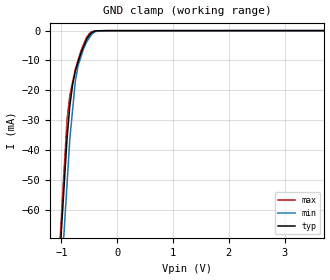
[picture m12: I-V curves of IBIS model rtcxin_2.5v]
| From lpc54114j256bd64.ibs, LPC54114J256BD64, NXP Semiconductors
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[Model] rtcxin_2.5v
Model_type Terminator
C_comp 1.70000pF 1.70000pF 1.70000pF
| variable typ   min   max
[Voltage Range] 2.50000V 2.25000V 2.75000V
[POWER Clamp Reference] 2.50000V 2.25000V 2.75000V
[GND Clamp Reference] 0.00000V 0.00000V 0.00000V
[Temperature Range]   25   85   -40
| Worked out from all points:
|   GND clamp passes 1 mA (typ) near -0.47 V on its own axis
[GND Clamp]
-2.5V     -525.9mA   -537.7mA   -545.3mA
-900mV    -36.15mA   -51.55mA   -29.8mA
-850mV    -25.2mA    -36.36mA   -21.71mA
-800mV    -18.11mA   -26.54mA   -17.27mA
-750mV    -13.44mA   -16.72mA   -12.84mA
-700mV    -10.44mA   -11.61mA   -9.774mA
-600mV    -5.193mA   -5.905mA   -4.474mA
-550mV    -2.953mA   -3.803mA   -2.235mA
-450mV    -591.7uA   -1.075mA   -286.4uA
-350mV    -34.81uA   -121.5uA   -43.27uA
-175mV    -6.375uA   -7.464uA   -2.304uA
5V        12.65uA    21.84uA    13.5uA
[POWER Clamp]
-2.5V     0A         0A         0A
5V        0A         0A         0A
